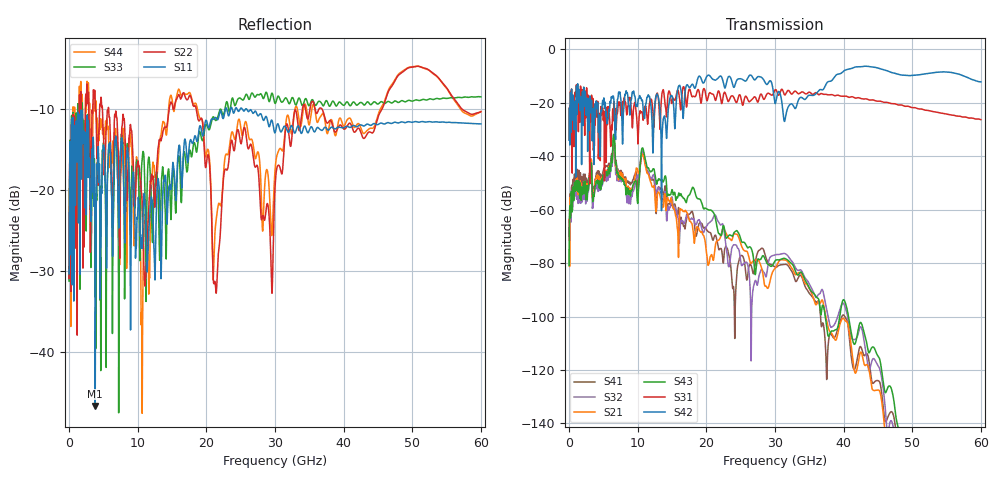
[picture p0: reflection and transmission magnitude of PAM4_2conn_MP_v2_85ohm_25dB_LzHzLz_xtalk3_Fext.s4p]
! Info: Touchstone file created by Circ.  Input file=FAB50GbE_2conn_Midplane_Examax_Topo2_v2_85ohm_25dB_LzHzLz.circ
# Hz S RI R 50
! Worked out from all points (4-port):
!   6000 points, 10 MHz to 60 GHz, reference 50 ohm
!   strongest paths, dB at 10 MHz, 15.01 GHz, 30.01 GHz, 45.01 GHz, 60 GHz:
!     S42: -34.0, -17.4, -20.2, -7.0, -12.1
!     S31: -33.8, -20.0, -15.1, -19.3, -26.3
!     S43: -80.9, -52.5, -79.2, -114.8, -171.0
!     S21: -63.6, -57.5, -82.0, -127.5, -173.6
!     S32: -67.4, -55.2, -76.9, -118.4, -165.8
!     S41: -66.9, -58.0, -81.5, -124.0, -184.0
!   lowest |S11| = -46.6 dB at 3.81 GHz (marker M1), VSWR 1.01, Z = 49.9 + j0.442 ohm
!   |S11| at or under -10 dB: start of sweep to 22.77 GHz; 22.99 GHz to 23.51 GHz (515 MHz wide, 2.22 % of centre); 25.91 GHz to end of sweep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
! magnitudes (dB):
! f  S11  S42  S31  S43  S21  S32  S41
! 10 MHz  -30.3  -34.0  -33.8  -80.9  -63.6  -67.4  -66.9
! 800 MHz  -12.1  -25.5  -17.7  -49.8  -51.2  -55.0  -46.8
! 3.81 GHz  -46.6  -24.4  -28.3  -51.1  -49.4  -52.3  -48.5
! 10.63 GHz  -26.6  -19.0  -23.4  -37.0  -39.2  -38.0  -38.1
! 14.77 GHz  -19.8  -17.7  -17.2  -54.4  -56.4  -58.7  -58.2
! 20.35 GHz  -12.3  -9.6  -16.8  -60.1  -80.4  -65.1  -68.3
! 60 GHz  -11.8  -12.1  -26.3  -171.0  -173.6  -165.8  -184.0
